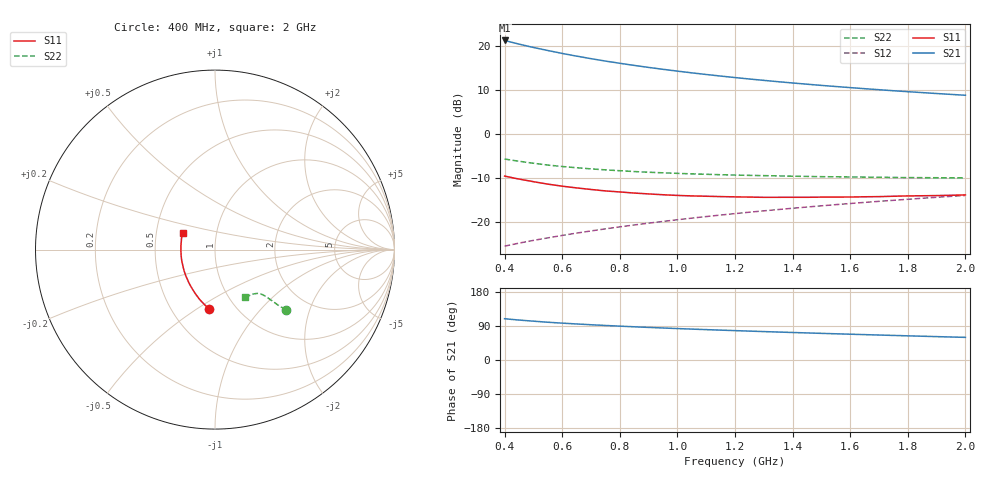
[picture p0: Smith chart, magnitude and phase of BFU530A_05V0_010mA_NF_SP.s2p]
! Filename:  P:\Prog\Test\Noise\ATS_data\Testdata_Net\06 Compressed Noise after Statistics\BFU530A_APG2013_33_A05_05p0V_010mA_NF_CM01_D.sf
! Date/Time: Tue 16/Apr/2013 15:10:59
! BFU530A_APG2013_33_A05_05p0V_1to25mA_NF_CM01_Bias5_R.sf
! Noise Parameter Data File
! BFU530A_APG2013_33_A05_05p0V_1to25mA_NF_CM01
! Date/time: Fri Apr 12 15:27:54 2013
! VAR V_out= 5.001000
! VAR I_out= 10.000000
! VAR V_in= 0.831700
! VAR I_in= 0.107205
! Device data file deembeded for feedlines and parallel
! Original file: \06 Compressed Noise after Statistics\BFU530A_APG2013_33_A05_05p0V_010mA_NF_CM01_R.sf
! Feed-files: PR017V01_150413_Feed1.s2p, PR017V01_150413_Feed2.s2p
! Parallel-file: PR017V01_150413_Par.s2p
# MHz S MA R 50
!  Freq-MHz  S11-mag  S11-arg  S21-mag  S21-arg  S12-mag  S12-arg  S22-mag  S22-arg
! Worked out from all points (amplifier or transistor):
!   37 points, 400 MHz to 2 GHz, reference 50 ohm
!   highest |S21| = 21.2 dB at 400 MHz (marker M1)
!   |S21| within 3 dB of that: start of sweep to 604.5 MHz
!   unconditionally stable (mu >= 1): 1.295 GHz to end of sweep
!   at 500 MHz: K = 0.81, MSG = 21.9 dB, |S12| = -24.2 dB
!   at 1.1 GHz: K = 0.99, MSG = 16.1 dB, |S12| = -18.8 dB
!   at 2 GHz: K = 1.01, MAG = 10.8 dB, |S12| = -14.0 dB
!   lowest NFmin = 0.77 dB at 420 MHz
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400  0.3308 -95.8  11.46 108.9  0.05301 64.8  0.5172 -40.3
420  0.3211 -98.5  11.02 107.5  0.05477 64.9  0.5043 -40.6
440  0.3108 -101.1  10.61 106.1  0.0565 65.0  0.4929 -40.8
460  0.302 -103.5  10.23 104.8  0.05825 65.1  0.4826 -41.1
480  0.2941 -106.0  9.872 103.6  0.05993 65.2  0.4721 -41.3
500  0.286 -108.5  9.538 102.5  0.06166 65.3  0.4632 -41.4
550  0.2682 -114.3  8.81 99.7  0.06583 65.7  0.4413 -41.7
600  0.2542 -119.4  8.161 97.3  0.07021 66.1  0.4252 -41.9
650  0.2429 -124.5  7.606 95.1  0.07459 66.3  0.4116 -42.2
700  0.2333 -129.2  7.118 93.0  0.07893 66.7  0.3997 -42.4
750  0.2246 -133.8  6.686 91.1  0.08336 66.9  0.3892 -42.5
800  0.2187 -138.1  6.309 89.3  0.0878 67.1  0.3808 -42.8
850  0.2124 -142.5  5.969 87.6  0.09224 67.3  0.3727 -43.1
950  0.2032 -150.4  5.39 84.5  0.1012 67.6  0.3605 -43.8
1050  0.1971 -157.7  4.913 81.5  0.1103 67.7  0.3507 -44.5
1150  0.1937 -164.6  4.517 78.8  0.1195 67.7  0.3429 -45.4
1200  0.1923 -167.8  4.344 77.5  0.1242 67.6  0.34 -45.9
1350  0.1901 -176.8  3.898 73.8  0.1381 67.3  0.3326 -47.6
1500  0.191 175.0  3.54 70.3  0.1521 66.9  0.3259 -49.5
1650  0.1928 167.8  3.248 67.0  0.1664 66.2  0.3222 -51.8
1750  0.1955 163.2  3.08 64.8  0.1757 65.8  0.3194 -53.3
2000  0.2024 153.3  2.736 59.7  0.1996 64.4  0.3157 -57.6
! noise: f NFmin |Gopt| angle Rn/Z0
400  0.8007  0.05815  172.8  0.0901
460  0.7749  0.06377  175.4  0.0863
600  0.8855  0.02995  -172.5  0.1024
800  0.8401  0.1024  -176.2  0.0836
1000  0.8622  0.1131  -172.1  0.0812
1200  0.9068  0.1302  -172.3  0.0817
1400  0.9139  0.1648  -163.7  0.0819
1600  0.9307  0.1878  -157.3  0.0786
1800  0.9263  0.227  -153.6  0.0724
2000  0.951  0.2492  -148.2  0.0748
